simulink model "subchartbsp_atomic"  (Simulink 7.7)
settings: Solver=ode1  StartTime=0.0  StopTime=1000  FixedStep=0.0001  RelTol=1e-3
libraries: simulink x4

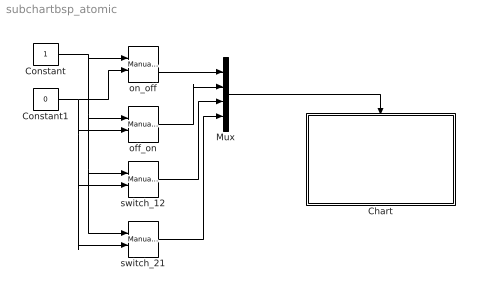
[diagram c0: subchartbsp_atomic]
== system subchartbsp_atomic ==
  Chart : Stateflow chart  TreatAsAtomicUnit=on
  Constant : Constant
  Constant1 : Constant  Value=0
  Mux : Mux
  off_on : simulink/Signal Routing/Manual Switch  SystemSampleTime=-1  sw=1  action=0  varsize=off
  on_off : simulink/Signal Routing/Manual Switch  SystemSampleTime=-1  sw=0  action=0  varsize=off
  switch_12 : simulink/Signal Routing/Manual Switch  SystemSampleTime=-1  sw=1  action=0  varsize=off
  switch_21 : simulink/Signal Routing/Manual Switch  SystemSampleTime=-1  sw=0  action=0  varsize=off
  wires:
  Constant1/1 -> on_off/2, off_on/2, switch_12/2, switch_21/2
  Constant/1 -> on_off/1, off_on/1, switch_12/1, switch_21/1
  on_off/1 -> Mux/1
  off_on/1 -> Mux/2
  switch_12/1 -> Mux/3
  switch_21/1 -> Mux/4
  Mux/1 -> Chart/Trigger

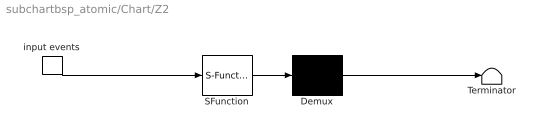
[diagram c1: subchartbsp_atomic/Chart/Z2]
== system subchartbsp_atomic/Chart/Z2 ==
  " input events " : TriggerPort  TriggerType=either  ShowOutputPort=on
  " Demux " : Demux  Outputs=1
  " SFunction " : S-Function  Tag=Stateflow S-Function subchartbsp_atomic 1  FunctionName=sf_sfun  PortCounts=[1 1]  EnableBusSupport=off
  " Terminator " : Terminator
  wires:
  " input events "/1 -> " SFunction "/1
  " Demux "/1 -> " Terminator "/1
  " SFunction "/1 -> " Demux "/1

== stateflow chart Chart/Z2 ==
  state Off
  state On
  On -> Off : on_off
  Off -> On : off_on
  (default) -> Off

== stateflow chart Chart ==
  state Z1
    state On
    state Off
    On -> Off : on_off
    Off -> On : off_on
    (default) -> On
  state Z2
  (default) -> Z1
  Z1 -> Z2 : switch_12
  Z2 -> Z1 : switch_21
